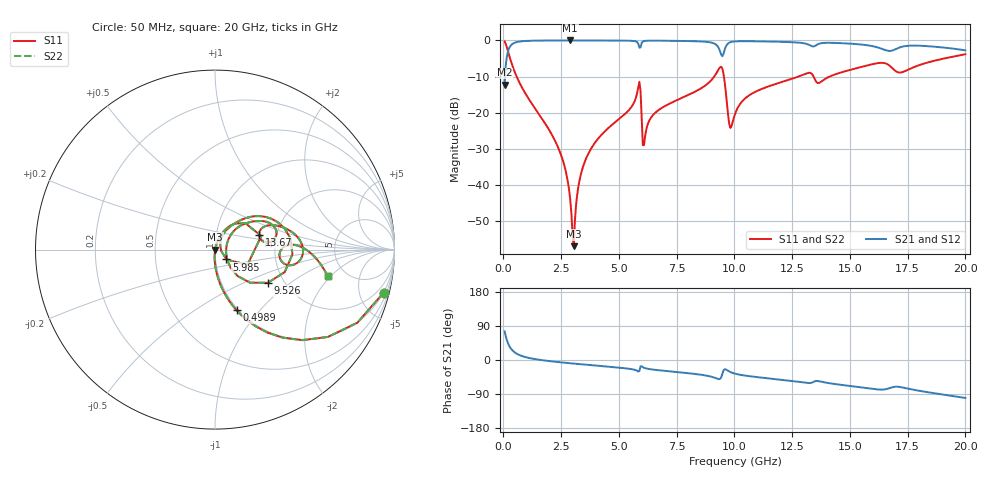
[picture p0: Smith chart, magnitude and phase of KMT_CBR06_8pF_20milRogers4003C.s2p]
! Data measured by Modelithics Inc. support@modelithics.com 813-866-6335
! KEMET CBR0603 8pF, Pad Width= 0.851mm, Pad Length= 0.64mm, Pad Gap= 0.62mm, 20mil Rogers 4003C substrate Data, January 2022
# hz S ma R 50
! 2 Port Network Data from SP1.SP block
! freq  magS11  angS11  magS21  angS21  magS12  angS12  magS22  angS22
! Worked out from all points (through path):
!   401 points, 50 MHz to 20 GHz, reference 50 ohm
!   highest |S21| = -0.01 dB at 2.893 GHz (marker M1); lowest = -12.2 dB at 50 MHz (marker M2)
!   group delay of S21, straight-line fit = 14.7 ps
!   lowest |S11| = -56.8 dB at 3.042 GHz (marker M3), VSWR 1.00, Z = 50.1 + j0.0467 ohm
!   |S11| at or under -10 dB: 571.7 MHz to 9.123 GHz (8.552 GHz wide, 176 % of centre); 9.545 GHz to 12.76 GHz (3.218 GHz wide, 28.9 % of centre); 13.43 GHz to 14.12 GHz (689.2 MHz wide, 5 % of centre)
!   |S22| runs from -56.8 to -0.3 dB; largest |S21 - S12| = 0
!   S11 on the Smith chart (normalised r, x): 50 MHz: 0.98, -7.81; 498.9 MHz: 0.98, -0.76; 5.985 GHz: 1.13, -0.13; 9.526 GHz: 1.65, -0.70; 13.67 GHz: 1.62, +0.29; 20 GHz: 3.63, -1.84
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5e7  0.9693 -14.4  0.2456 75.6  0.2456 75.6  0.9693 -14.4
2.495e8  0.6175 -52.6  0.7857 37.4  0.7857 37.4  0.6175 -52.6
4.98875e8  0.3593 -70.4  0.9324 19.5  0.9324 19.5  0.3593 -70.4
2.394125e9  0.03169 -93.6  0.9983 -5.6  0.9983 -5.6  0.03169 -93.6
2.693375e9  0.01584 -93.1  0.9986 -7.4  0.9986 -7.4  0.01584 -93.1
2.892875e9  0.006284 -87.3  0.9986 -8.6  0.9986 -8.6  0.006284 -87.3
3.0425e9  0.001441 18.9  0.9986 -9.5  0.9986 -9.5  0.001441 18.9
3.391625e9  0.01578 73.7  0.9984 -11.4  0.9984 -11.4  0.01578 73.7
3.94025e9  0.0378 73.4  0.9977 -14.4  0.9977 -14.4  0.0378 73.4
5.8355e9  0.2238 41.3  0.9062 -30.3  0.9062 -30.3  0.2238 41.3
5.985125e9  0.08426 -40.8  0.9224 -16.5  0.9224 -16.5  0.08426 -40.8
6.13475e9  0.04813 52.0  0.9851 -21.6  0.9851 -21.6  0.04813 52.0
6.73325e9  0.1101 61.2  0.9904 -27.1  0.9904 -27.1  0.1101 61.2
9.12725e9  0.3175 35.8  0.9058 -46.4  0.9058 -46.4  0.3175 35.8
9.52625e9  0.3475 -32.2  0.6528 -27.7  0.6528 -27.7  0.3475 -32.2
9.775625e9  0.06979 -25.6  0.9301 -30.3  0.9301 -30.3  0.06979 -25.6
1.0025e10  0.09589 37.9  0.9689 -36.0  0.9689 -36.0  0.09589 37.9
1.087288e10  0.1928 43.2  0.9729 -44.4  0.9729 -44.4  0.1928 43.2
1.336662e10  0.3409 10.5  0.83 -59.4  0.83 -59.4  0.3409 10.5
1.366588e10  0.2589 18.6  0.8993 -56.1  0.8993 -56.1  0.2589 18.6
1.670825e10  0.4505 -10.6  0.7153 -74.4  0.7153 -74.4  0.4505 -10.6
2e10  0.6443 -13.3  0.7295 -100.2  0.7295 -100.2  0.6443 -13.3
